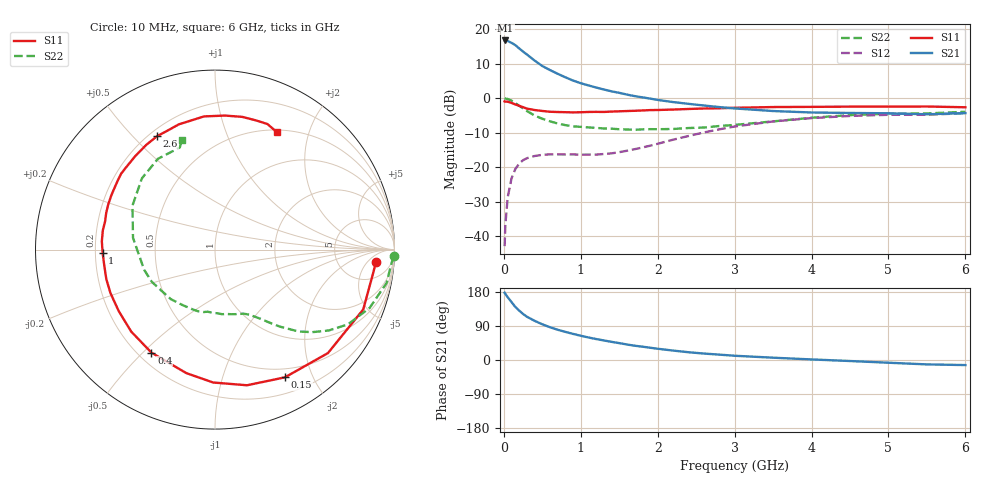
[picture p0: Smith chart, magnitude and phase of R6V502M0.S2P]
! SIEMENS Small Signal Semiconductors
! BFR193
! Si NPN RF Bipolar Junction Transistor in SOT23
! VCE = 0.5 V  IC = 2 mA
! Common Emitter S-Parameters:  May  1996
# GHz  S  MA  R  50
!  f  S11  S21  S12  S22
! GHz  MAG  ANG  MAG  ANG  MAG  ANG  MAG  ANG
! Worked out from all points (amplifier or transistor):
!   36 points, 10 MHz to 6 GHz, reference 50 ohm
!   highest |S21| = 16.7 dB at 20 MHz (marker M1)
!   |S21| within 3 dB of that: start of sweep to 237.5 MHz
!   unconditionally stable (mu >= 1): 1.115 GHz to 2.407 GHz; 4.799 GHz to end of sweep
!   at 250 MHz: K = 0.25, MSG = 15.7 dB, |S12| = -17.9 dB
!   at 1.4 GHz: K = 1.15, MAG = 6.6 dB, |S12| = -16.0 dB
!   at 6 GHz: K = 1.01, MAG = -0.7 dB, |S12| = -4.3 dB
!   S11 on the Smith chart (normalised r, x): 10 MHz: 12, -9; 150 MHz: 0.39, -1.62; 400 MHz: 0.25, -0.53; 1 GHz: 0.23, -0.01; 2.6 GHz: 0.23, +0.59; 6 GHz: 0.53, +1.53
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0.01  0.8996 -4.5  6.753 177.5  0.0072 86.5  0.996 -2.2
0.02  0.8905 -8.6  6.858 174.2  0.0148 85.0  0.9863 -4.4
0.05  0.8907 -22.0  6.744 165.9  0.0366 77.2  0.9742 -11.0
0.1  0.8535 -42.5  6.332 152.7  0.0692 67.0  0.9207 -20.7
0.15  0.8114 -61.3  5.863 139.9  0.0945 57.1  0.8494 -29.4
0.2  0.7766 -76.7  5.256 130.3  0.1132 49.6  0.7777 -35.4
0.25  0.7406 -90.8  4.729 121.5  0.1267 43.7  0.7112 -40.3
0.3  0.7064 -103.1  4.291 114.2  0.1352 39.1  0.6521 -44.4
0.4  0.6744 -121.7  3.508 103.4  0.1455 32.4  0.5609 -49.9
0.5  0.6532 -135.6  2.926 94.2  0.1514 28.1  0.5042 -53.5
0.6  0.6365 -147.4  2.555 86.5  0.1538 25.7  0.4625 -56.6
0.7  0.6309 -157.4  2.257 79.8  0.1536 24.7  0.4301 -59.8
0.8  0.6274 -164.8  2.007 74.2  0.1531 24.6  0.407 -62.8
1  0.6262 -178.2  1.648 64.0  0.1522 25.8  0.3848 -68.6
1.1  0.6321 175.9  1.531 59.4  0.1526 27.6  0.3778 -72.2
1.6  0.6518 152.5  1.128 40.9  0.1733 41.0  0.3526 -92.2
2.2  0.685 130.3  0.879 24.9  0.2506 48.6  0.3584 -120.7
2.6  0.7094 117.1  0.784 17.0  0.3193 46.3  0.3761 -142.4
3.5  0.7446 94.7  0.652 6.1  0.4606 31.3  0.4616 171.8
4.5  0.7549 78.4  0.611 -2.7  0.5536 13.2  0.5689 135.7
5.5  0.7581 67.3  0.585 -11.6  0.5762 -2.6  0.6017 109.0
6  0.7392 62.1  0.608 -13.4  0.6062 -7.2  0.6361 107.0
